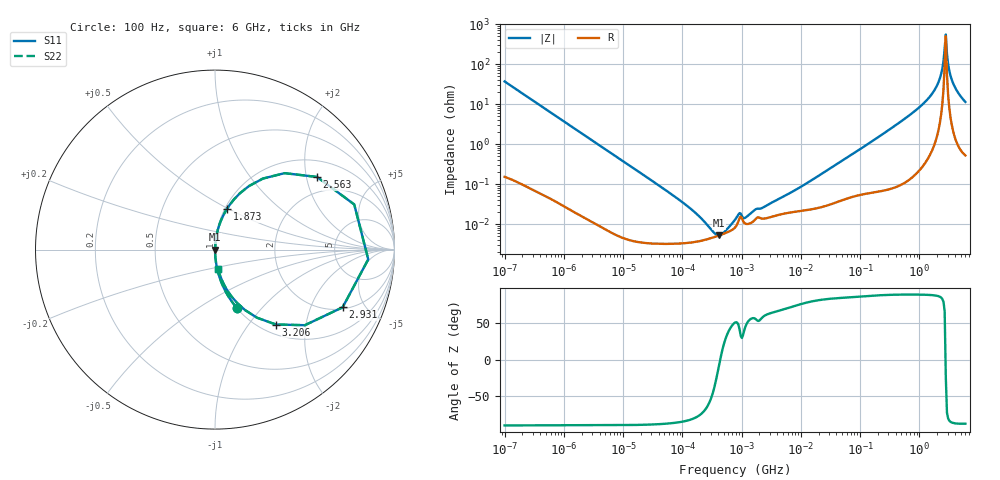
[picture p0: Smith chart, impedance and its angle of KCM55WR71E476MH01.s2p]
!Murata Part Number: KCM55WR71E476MH01
!These Parameters are Measured in Series Mode Connection
!Data Generated on Mar 13, 2026
!  o--ll--o
!Port1  Port2
!  o------o
!Operation Temp=25[degC], DC Bias Voltage=0[V]
!Freq. Start=100[Hz] Stop=6[GHz] 401[Steps]
# Hz S RI R 50
!Freq.(Hz) S11(Real) S11(Imag) S21(Real) S21(Imag) S12(Real) S12(Imag) S22(Real) S22(Imag)
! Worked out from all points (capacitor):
!   401 points, 100 Hz to 6 GHz, reference 50 ohm
!   read as one part in series: C = 43.1 uF near 109 Hz
!   lowest |Z| = 5.28 mohm at 413.8 kHz (marker M1)
!   series resonance near 436.2 kHz, so ESL is about 3.1 nH
!   S11 on the Smith chart (normalised r, x): 100 Hz: 1.00, -0.74; 1.873 GHz: 1.02, +0.49; 2.563 GHz: 1.47, +2.31; 2.931 GHz: 2.09, -3.44; 3.206 GHz: 1.16, -1.37; 6 GHz: 1.01, -0.23
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100  0.1205 -0.3235  0.8795 0.3235  0.8795 0.3235  0.1205 -0.3235
366  0.0107 -0.0999  0.9893 0.0999  0.9893 0.0999  0.0107 -0.0999
2008  0.000502 -0.0186  0.9995 0.0186  0.9995 0.0186  0.000502 -0.0186
40335  3.32e-05 -0.000923  1 0.000923  1 0.000923  3.32e-05 -0.000923
252896  4.13e-05 -9.42e-05  1 9.42e-05  1 9.42e-05  4.13e-05 -9.42e-05
413847  5.21e-05 -8.3e-06  0.9999 8.3e-06  0.9999 8.3e-06  5.21e-05 -8.3e-06
647581  6.82e-05 6.37e-05  0.9999 -6.37e-05  0.9999 -6.37e-05  6.82e-05 6.37e-05
774597  8.22e-05 9.93e-05  0.9999 -9.93e-05  0.9999 -9.93e-05  8.22e-05 9.93e-05
926525  0.000143 0.000124  0.9999 -0.000124  0.9999 -0.000124  0.000143 0.000124
1212075  0.000101 0.000114  0.9999 -0.000114  0.9999 -0.000114  0.000101 0.000114
1.555665e7  0.000238 0.00126  0.9998 -0.00126  0.9998 -0.00126  0.000238 0.00126
3.124326e8  0.00128 0.023  0.9987 -0.023  0.9987 -0.023  0.00128 0.023
1.046602e9  0.01 0.0871  0.99 -0.0871  0.99 -0.0871  0.01 0.0871
1.873145e9  0.0663 0.2263  0.9337 -0.2263  0.9337 -0.2263  0.0663 0.2263
2.142435e9  0.1395 0.3146  0.8605 -0.3146  0.8605 -0.3146  0.1395 0.3146
2.34314e9  0.2666 0.3957  0.7334 -0.3957  0.7334 -0.3957  0.2666 0.3957
2.562649e9  0.5687 0.4047  0.4313 -0.4047  0.4313 -0.4047  0.5687 0.4047
2.802721e9  0.8538 -0.0542  0.1462 0.0542  0.1462 0.0542  0.8538 -0.0542
2.931063e9  0.7111 -0.3215  0.2889 0.3215  0.2889 0.3215  0.7111 -0.3215
3.205649e9  0.3392 -0.4173  0.6608 0.4173  0.6608 0.4173  0.3392 -0.4173
3.8344e9  0.0956 -0.2657  0.9044 0.2657  0.9044 0.2657  0.0956 -0.2657
6e9  0.0176 -0.1103  0.9824 0.1103  0.9824 0.1103  0.0176 -0.1103
